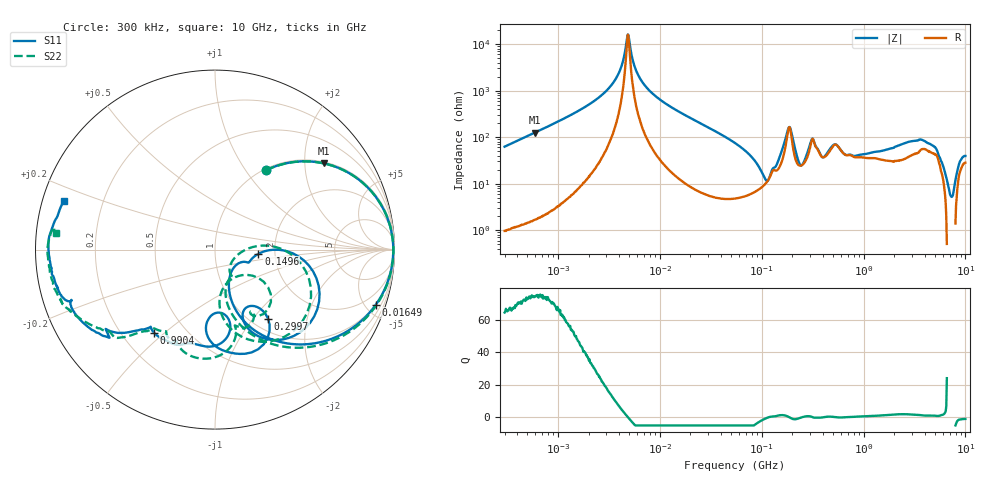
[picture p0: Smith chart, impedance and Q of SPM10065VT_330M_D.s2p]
! S-Parameter Data Generated by TDK Corporation
! Copyright(C) 2020 TDK Corporation.
! All Rights Reserved.
! TDK P/N: SPM10065VT-330M-D (Inductor)
! Property: L=33uH at 100kHz
! Size(LxWxT): 10.5x10x6.5mm
! Model Type: s2p (Touchstone File Format Version 1.0)
! Frequency: DC=Yes Start=0.3MHz Stop=10000MHz 802points Log-sweep
! Model Generated on Aug. 18, 2020
! Port Assignments:
!  1 ---@@@--- 2
! Applicable Conditions:
!  Temperature = 25 degC
!  DC Bias Current = 0 A
!  Small Signal Operation
! Terms and conditions regarding TDK Simulation Models
! (1)This simulation model is being provided solely for informational purposes. Please refer to the specifications of the products in terms of detailed characteristics of such products.
! (2)In no event shall TDK Corporation of any of its subsidiaries be liable for any loss or damage arising, directly or indirectly,
!  From any information contained in this simulation model, including, but not limited to loss or damages arising from any inaccuracies, omissions or errors in connection with such information.
! (3)Any and all copyrights on this simulation model are owned by TDK Corporation.
!  Duplication or redistribution of this simulation model without prior written permission from TDK Corporation is prohibited.
! (4)This simulation model is subject to any modification or change without any prior notice.
! (5)Neither TDK Corporation nor any of its subsidiaries shall make any warranty, express or implied,
!  Including but not limited to the correctness, implied warranties of merchantability and fitness for a particular purpose with respect to this simulation models.
! (6)The use of this simulation model shall be deemed to have consented to the terms and conditions hereof.
# Hz S MA R 50
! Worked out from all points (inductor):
!   801 points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, 300 kHz to 10 GHz, reference 50 ohm
!   read as one part in series: L = 33 uH near 318.3 kHz
!   highest Q = 74.5 at 592.8 kHz (marker M1), where L = 33.4 uH
!   self-resonance near 4.859 MHz
!   S11 on the Smith chart (normalised r, x): 300 kHz: 1.02, +1.25; 16.49 MHz: 0.98, -5.82; 149.6 MHz: 1.64, -0.08; 299.7 MHz: 1.19, -1.19; 990.4 MHz: 0.33, -0.46; 10 GHz: 0.06, +0.16
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300000  0.5263 57.3  0.8429 -31.8  0.8422 -31.9  0.5256 57.3
592755  0.7737 38.4  0.6219 -50.9  0.6218 -50.9  0.7739 38.4
1713600  0.9647 13.6  0.2391 -75.1  0.2391 -75.1  0.9653 13.5
3553821  0.9918 3.2  0.06355 -81.8  0.06355 -81.8  0.9923 3.0
4858855  0.9934 -0.6  0.006174 -8.5  0.006177 -9.1  0.994 -0.8
6298968  0.9916 -3.7  0.05107 78.7  0.0511 78.8  0.9921 -4.0
9671944  0.9817 -9.5  0.1436 77.2  0.1435 77.2  0.9821 -10.0
1.649435e7  0.9467 -19.0  0.2896 68.6  0.2896 68.6  0.947 -19.8
5.477226e7  0.6203 -55.5  0.7491 29.7  0.7489 29.7  0.6195 -58.4
1.210198e8  0.1476 -48.4  0.8618 -13.0  0.8616 -13.0  0.1788 -60.3
1.495617e8  0.2432 -5.5  0.8023 -27.0  0.8021 -27.0  0.1641 -1.3
1.900804e8  0.6665 -34.0  0.3639 -15.2  0.3638 -15.2  0.6296 -39.2
2.351426e8  0.4341 -68.2  0.7366 -16.2  0.7364 -16.2  0.3443 -84.8
2.694285e8  0.3686 -58.8  0.7254 -33.4  0.7252 -33.4  0.1906 -64.2
2.996953e8  0.4854 -52.5  0.569 -45.7  0.5688 -45.7  0.3247 -33.4
3.126428e8  0.5729 -59.2  0.4682 -41.7  0.468 -41.7  0.4272 -43.2
3.7738e8  0.4723 -95.6  0.5913 -29.3  0.5912 -29.3  0.4639 -66.1
5.82867e8  0.5411 -97.1  0.4635 -50.0  0.4634 -50.0  0.6097 -94.4
9.903836e8  0.5745 -126.3  0.4285 -85.1  0.4285 -85.1  0.5447 -123.7
1.767019e9  0.6963 -138.2  0.2333 -146.2  0.2332 -146.2  0.6865 -135.3
4.924213e9  0.9102 -168.9  0.02242 -168.6  0.02244 -168.4  0.9124 -164.1
1e10  0.8825 162.1  0.02949 143.6  0.02954 143.5  0.8928 174.1
